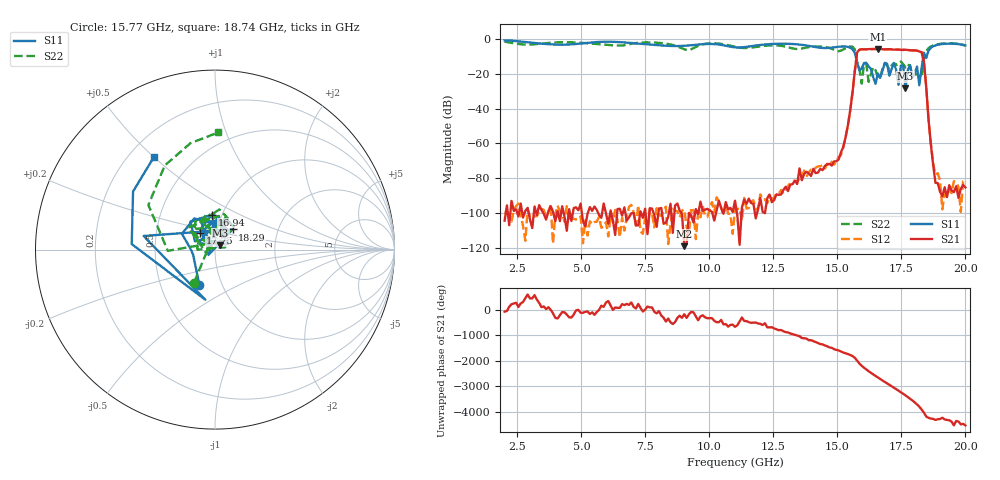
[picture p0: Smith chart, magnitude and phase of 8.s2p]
!Keysight Technologies,N5234A,MY52241180,A.10.60.03
!Date: Friday, January 20, 2023 09:34:49
!Correction: S11(Full 2 Port(1,2))
!S21(Full 2 Port(1,2))
!S12(Full 2 Port(1,2))
!S22(Full 2 Port(1,2))
!S2P File: Measurements: S11, S21, S12, S22:
# Hz S  dB  R 50
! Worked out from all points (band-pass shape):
!   201 points, 2 GHz to 20 GHz, reference 50 ohm
!   highest |S21| = -5.67 dB at 16.58 GHz (marker M1); lowest = -119.0 dB at 9.02 GHz (marker M2)
!   |S21| within 3 dB of the highest: 15.76 GHz to 18.31 GHz (2.546 GHz wide, 14.9 % of centre)
!   lowest |S11| = -28.3 dB at 17.66 GHz (marker M3), VSWR 1.08, Z = 53 + j2.6 ohm
!   |S11| at or under -10 dB: 15.71 GHz to 18.36 GHz (2.643 GHz wide, 15.5 % of centre); 18.44314 GHz to 18.48929 GHz (46.15 MHz wide, 0.25 % of centre)
!   |S22| runs from -25.6 to -1.5 dB; largest |S21 - S12| = 0.00066
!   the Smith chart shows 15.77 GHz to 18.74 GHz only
!   S11 on the Smith chart (normalised r, x): 15.77 GHz: 0.78, -0.32; 16.94 GHz: 0.90, +0.36; 17.75 GHz: 0.83, +0.16; 18.29 GHz: 1.18, +0.27; 18.74 GHz: 0.30, +0.50
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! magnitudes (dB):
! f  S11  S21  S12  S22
! 2 GHz  -0.8  -104.4  -99.4  -1.5
! 5.06 GHz  -2.4  -104.7  -117.4  -2.2
! 8.03 GHz  -3.6  -97.4  -101.3  -2.2
! 9.02 GHz  -3.9  -119.0  -97.9  -5.9
! 11 GHz  -4.8  -92.9  -97.3  -4.4
! 14.06 GHz  -4.4  -74.6  -75.4  -4.3
! 15.14 GHz  -4.3  -65.1  -66.7  -6.7
! 15.41 GHz  -4.5  -49.6  -49.7  -4.7
! 15.77 GHz  -13.4  -7.7  -7.7  -13.2
! 15.95 GHz  -17.0  -5.9  -5.9  -25.6
! 16.04 GHz  -13.8  -5.9  -5.9  -14.3
! 16.58 GHz  -19.7  -5.7  -5.7  -22.2
! 16.94 GHz  -14.2  -5.9  -5.9  -15.1
! 17.03 GHz  -21.0  -5.8  -5.8  -17.7
! 17.57 GHz  -15.4  -6.2  -6.2  -14.5
! 17.66 GHz  -28.3  -6.2  -6.2  -16.3
! 17.75 GHz  -18.0  -6.3  -6.3  -14.5
! 18.11 GHz  -15.8  -6.7  -6.7  -20.2
! 18.2 GHz  -26.5  -7.1  -7.1  -21.4
! 18.29 GHz  -16.5  -7.6  -7.6  -21.7
! 18.74 GHz  -4.2  -72.2  -71.5  -3.7
! 20 GHz  -3.7  -85.3  -81.1  -3.9
